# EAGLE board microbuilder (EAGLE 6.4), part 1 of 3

Size 273.6 x 738.6 mm. Coordinates in mm from the lower left corner, seen from the top.
Copper layers (1*16): Top 0.035mm / dielectric 1.5mm / Bottom 0.035mm
Design rules "default": minimum track width 10mil, minimum drill 24mil, track to track 8mil, track to pad 8mil, pad to pad 8mil, via to via 8mil, smd to smd 8mil, copper to edge 40mil, drill to drill 8mil, minimum pad ring 10mil, minimum via ring 8mil, stop-mask expansion 4mil, vias tented up to drill 0mil, thermal gap 10mil

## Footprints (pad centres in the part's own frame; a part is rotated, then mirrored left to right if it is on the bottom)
1X01_2MM = drill 0.8 pad 1.27: 1 0,0
1X01_2MM_OVAL = drill 0.8 pad 1.27 long: 1 0,0
1X01_OVAL = drill 1 pad 1.676 long: 1 0,0
1X01_ROUND = drill 1 pad 1.676: 1 0,0
1X02_OVAL = drill 1 long: 1 -1.27,0; 2 1.27,0
1X02_ROUND = drill 1 pad 1.676: 1 -1.27,0; 2 1.27,0
1X02_SMT = smd 1 x 3.5: 1 -1.27,1.27; 2 1.27,-1.27
1X03_1.0MM = smd 0.5 x 2.5: 1 -1,0; 2 0,0; 3 1,0
1X03_OVAL = drill 1 long: 1 -2.54,0; 2 0,0; 3 2.54,0
1X03_ROUND = drill 1 pad 1.676: 1 -2.54,0; 2 0,0; 3 2.54,0
1X03_ROUND_76 = drill 1 pad 1.93: 1 -2.54,0; 2 0,0; 3 2.54,0
1X03_SMT = smd 1 x 3.5: 1 -2.54,1.27; 2 0,-1.27; 3 2.54,1.27
1X04_1.0MM = smd 0.5 x 2.5: 1 -2,0; 2 -1,0; 3 0,0; 4 1,0
1X04_OVAL = drill 1 long: 1 -3.81,0; 2 -1.27,0; 3 1.27,0; 4 3.81,0
1X04_ROUND = drill 1 pad 1.676: 1 -3.81,0; 2 -1.27,0; 3 1.27,0; 4 3.81,0
1X04_ROUND_76 = drill 1 pad 1.93: 1 -3.81,0; 2 -1.27,0; 3 1.27,0; 4 3.81,0
1X04_SMT = smd 1 x 3: 1 -3.81,1.27; 2 -1.27,-1.27; 3 1.27,1.27; 4 3.81,-1.27
1X05_1.27MM = smd 0.5 x 2.5: 1 -2.54,0; 2 -1.27,0; 3 0,0; 4 1.27,0; 5 2.54,0
1X05_OVAL = drill 1 long: 1 -5.08,0; 2 -2.54,0; 3 0,0; 4 2.54,0; 5 5.08,0
1X05_ROUND = drill 1 pad 1.676: 1 -5.08,0; 2 -2.54,0; 3 0,0; 4 2.54,0; 5 5.08,0
1X05_ROUND_70 = drill 1 pad 1.778: 1 -5.08,0; 2 -2.54,0; 3 0,0; 4 2.54,0; 5 5.08,0
1X05_ROUND_76 = drill 1 pad 1.93: 1 -5.08,0; 2 -2.54,0; 3 0,0; 4 2.54,0; 5 5.08,0
1X05_SMT = smd 1 x 3.5: 1 -5.08,1.27; 2 -2.54,-1.27; 3 0,1.27; 4 2.54,-1.27; 5 5.08,1.27
1X06_OVAL = drill 1 long: 1 -6.35,0; 2 -3.81,0; 3 -1.27,0; 4 1.27,0; 5 3.81,0; 6 6.35,0
1X06_ROUND = drill 1 pad 1.676: 1 -6.35,0; 2 -3.81,0; 3 -1.27,0; 4 1.27,0; 5 3.81,0; 6 6.35,0
1X06_ROUND_70 = drill 1 pad 1.778: 1 -6.35,0; 2 -3.81,0; 3 -1.27,0; 4 1.27,0; 5 3.81,0; 6 6.35,0
1X06_ROUND_76 = drill 1 pad 1.93: 1 -6.35,0; 2 -3.81,0; 3 -1.27,0; 4 1.27,0; 5 3.81,0; 6 6.35,0
1X06_SMT = smd 1 x 3.5: 1 -6.35,1.27; 2 -3.81,-1.27; 3 -1.27,1.27; 4 1.27,-1.27; 5 3.81,1.27; 6 6.35,-1.27
1X07_OVAL = drill 1 long: 1 -7.62,0; 2 -5.08,0; 3 -2.54,0; 4 0,0; 5 2.54,0; 6 5.08,0; 7 7.62,0
1X07_ROUND = drill 1 pad 1.676: 1 -7.62,0; 2 -5.08,0; 3 -2.54,0; 4 0,0; 5 2.54,0; 6 5.08,0; 7 7.62,0
1X07_ROUND_70 = drill 1 pad 1.778: 1 -7.62,0; 2 -5.08,0; 3 -2.54,0; 4 0,0; 5 2.54,0; 6 5.08,0; 7 7.62,0
1X07_ROUND_76 = drill 1 pad 1.93: 1 -7.62,0; 2 -5.08,0; 3 -2.54,0; 4 0,0; 5 2.54,0; 6 5.08,0; 7 7.62,0
1X08_OVAL = drill 1 long: 1 -8.89,0; 2 -6.35,0; 3 -3.81,0; 4 -1.27,0; 5 1.27,0; 6 3.81,0; 7 6.35,0; 8 8.89,0
1X08_ROUND = drill 1 pad 1.676: 1 -8.89,0; 2 -6.35,0; 3 -3.81,0; 4 -1.27,0; 5 1.27,0; 6 3.81,0; 7 6.35,0; 8 8.89,0
1X08_ROUND_70 = drill 1 pad 1.778: 1 -8.89,0; 2 -6.35,0; 3 -3.81,0; 4 -1.27,0; 5 1.27,0; 6 3.81,0; 7 6.35,0; 8 8.89,0
1X08_ROUND_76 = drill 1 pad 1.93: 1 -8.89,0; 2 -6.35,0; 3 -3.81,0; 4 -1.27,0; 5 1.27,0; 6 3.81,0; 7 6.35,0; 8 8.89,0
1X09_OVAL = drill 1 long: 1 -10.16,0; 2 -7.62,0; 3 -5.08,0; 4 -2.54,0; 5 0,0; 6 2.54,0; 7 5.08,0; 8 7.62,0; 9 10.16,0
1X09_ROUND_70 = drill 1 pad 1.778: 1 -10.16,0; 2 -7.62,0; 3 -5.08,0; 4 -2.54,0; 5 0,0; 6 2.54,0; 7 5.08,0; 8 7.62,0; 9 10.16,0
1X09_ROUND_76 = drill 1 pad 1.93: 1 -10.16,0; 2 -7.62,0; 3 -5.08,0; 4 -2.54,0; 5 0,0; 6 2.54,0; 7 5.08,0; 8 7.62,0; 9 10.16,0
1X10_OVAL = drill 1 long: 1 -11.43,0; 2 -8.89,0; 3 -6.35,0; 4 -3.81,0; 5 -1.27,0; 6 1.27,0; 7 3.81,0; 8 6.35,0; 9 8.89,0; 10 11.43,0
1X10_ROUND = drill 1 pad 1.676: 1 -11.43,0; 2 -8.89,0; 3 -6.35,0; 4 -3.81,0; 5 -1.27,0; 6 1.27,0; 7 3.81,0; 8 6.35,0; 9 8.89,0; 10 11.43,0
1X10_ROUND70 = drill 1 pad 1.778: 1 -11.43,0; 2 -8.89,0; 3 -6.35,0; 4 -3.81,0; 5 -1.27,0; 6 1.27,0; 7 3.81,0; 8 6.35,0; 9 8.89,0; 10 11.43,0
1X10_ROUND_2MM = drill 1 pad 1.5: 1 -10,0; 2 -8,0; 3 -6,0; 4 -4,0; 5 -2,0; 6 0,0; 7 2,0; 8 4,0; 9 6,0; 10 8,0
1X10_ROUND_76 = drill 1 pad 1.93: 1 -11.43,0; 2 -8.89,0; 3 -6.35,0; 4 -3.81,0; 5 -1.27,0; 6 1.27,0; 7 3.81,0; 8 6.35,0; 9 8.89,0; 10 11.43,0
1X10_SMT = smd 1 x 3.5: 1 -11.43,1.27; 2 -8.89,-1.27; 3 -6.35,1.27; 4 -3.81,-1.27; 5 -1.27,1.27; 6 1.27,-1.27; 7 3.81,1.27; 8 6.35,-1.27; 9 8.89,1.27; 10 11.43,-1.27
1X11_ROUND = drill 1 pad 1.676: 1 -12.7,0; 2 -10.16,0; 3 -7.62,0; 4 -5.08,0; 5 -2.54,0; 6 0,0; 7 2.54,0; 8 5.08,0; 9 7.62,0; 10 10.16,0; 11 12.7,0
1X11_ROUND_76 = drill 1 pad 1.93: 1 -12.7,0; 2 -10.16,0; 3 -7.62,0; 4 -5.08,0; 5 -2.54,0; 6 0,0; 7 2.54,0; 8 5.08,0; 9 7.62,0; 10 10.16,0; 11 12.7,0
1X12_OVAL = drill 1 pad 1.676 long: 1 -13.97,0; 2 -11.43,0; 3 -8.89,0; 4 -6.35,0; 5 -3.81,0; 6 -1.27,0; 7 1.27,0; 8 3.81,0; 9 6.35,0; 10 8.89,0; 11 11.43,0; 12 13.97,0
1X12_ROUND = drill 1 pad 1.676: 1 -13.97,0; 2 -11.43,0; 3 -8.89,0; 4 -6.35,0; 5 -3.81,0; 6 -1.27,0; 7 1.27,0; 8 3.81,0; 9 6.35,0; 10 8.89,0; 11 11.43,0; 12 13.97,0
1X12_ROUND_76MIL = drill 1 pad 1.93: 1 -13.97,0; 2 -11.43,0; 3 -8.89,0; 4 -6.35,0; 5 -3.81,0; 6 -1.27,0; 7 1.27,0; 8 3.81,0; 9 6.35,0; 10 8.89,0; 11 11.43,0; 12 13.97,0
1X12_ROUND_80MIL = drill 1 pad 2.032: 1 -13.97,0; 2 -11.43,0; 3 -8.89,0; 4 -6.35,0; 5 -3.81,0; 6 -1.27,0; 7 1.27,0; 8 3.81,0; 9 6.35,0; 10 8.89,0; 11 11.43,0; 12 13.97,0
1X13_ROUND_70 = drill 1 pad 1.676: 1 -15.24,0; 2 -12.7,0; 3 -10.16,0; 4 -7.62,0; 5 -5.08,0; 6 -2.54,0; 7 0,0; 8 2.54,0; 9 5.08,0; 10 7.62,0; 11 10.16,0; 12 12.7,0; 13 15.24,0
1X15_ROUND_70 = drill 1 pad 1.676: 1 -17.78,0; 2 -15.24,0; 3 -12.7,0; 4 -10.16,0; 5 -7.62,0; 6 -5.08,0; 7 -2.54,0; 8 0,0; 9 2.54,0; 10 5.08,0; 11 7.62,0; 12 10.16,0; 13 12.7,0; 14 15.24,0; 15 17.78,0
1X16_2MM = drill 0.8 pad 1.27: P$1 -15,0; P$2 -13,0; P$3 -11,0; P$4 -9,0; P$5 -7,0; P$6 -5,0; P$7 -3,0; P$8 -1,0; P$9 1,0; P$10 3,0; P$11 5,0; P$12 7,0; P$13 9,0; P$14 11,0; P$15 13,0; P$16 15,0
1X16_2MM_OVAL = drill 0.8 pad 1.27 long: P$1 -15,0; P$2 -13,0; P$3 -11,0; P$4 -9,0; P$5 -7,0; P$6 -5,0; P$7 -3,0; P$8 -1,0; P$9 1,0; P$10 3,0; P$11 5,0; P$12 7,0; P$13 9,0; P$14 11,0; P$15 13,0; P$16 15,0
1X16_OVAL = drill 1 long: 1 -19.05,0; 2 -16.51,0; 3 -13.97,0; 4 -11.43,0; 5 -8.89,0; 6 -6.35,0; 7 -3.81,0; 8 -1.27,0; 9 1.27,0; 10 3.81,0; 11 6.35,0; 12 8.89,0; 13 11.43,0; 14 13.97,0; 15 16.51,0; 16 19.05,0
1X16_ROUND = drill 1 pad 1.676: 1 -19.05,0; 2 -16.51,0; 3 -13.97,0; 4 -11.43,0; 5 -8.89,0; 6 -6.35,0; 7 -3.81,0; 8 -1.27,0; 9 1.27,0; 10 3.81,0; 11 6.35,0; 12 8.89,0; 13 11.43,0; 14 13.97,0; 15 16.51,0; 16 19.05,0
1X17_ROUND70 = drill 1 pad 1.778: 1 -20.32,0; 2 -17.78,0; 3 -15.24,0; 4 -12.7,0; 5 -10.16,0; 6 -7.62,0; 7 -5.08,0; 8 -2.54,0; 9 0,0; 10 2.54,0; 11 5.08,0; 12 7.62,0; 13 10.16,0; 14 12.7,0; 15 15.24,0; 16 17.78,0; 17 20.32,0
1X20_ROUND = drill 1 pad 1.676: 1 -24.13,0; 2 -21.59,0; 3 -19.05,0; 4 -16.51,0; 5 -13.97,0; 6 -11.43,0; 7 -8.89,0; 8 -6.35,0; 9 -3.81,0; 10 -1.27,0; 11 1.27,0; 12 3.81,0; 13 6.35,0; 14 8.89,0; 15 11.43,0; 16 13.97,0; 17 16.51,0; 18 19.05,0; 19 21.59,0; 20 24.13,0
1X23_ROUND_70MIL = drill 1 pad 1.676: 1 -27.94,0; 2 -25.4,0; 3 -22.86,0; 4 -20.32,0; 5 -17.78,0; 6 -15.24,0; 7 -12.7,0; 8 -10.16,0; 9 -7.62,0; 10 -5.08,0; 11 -2.54,0; 12 0,0; 13 2.54,0; 14 5.08,0; 15 7.62,0; 16 10.16,0; 17 12.7,0; 18 15.24,0; 19 17.78,0; 20 20.32,0; 21 22.86,0; 22 25.4,0; 23 27.94,0
1X27_OVAL = drill 1 pad 1.676 long: 1 -34.29,0; 2 -31.75,0; 3 -29.21,0; 4 -26.67,0; 5 -24.13,0; 6 -21.59,0; 7 -19.05,0; 8 -16.51,0; 9 -13.97,0; 10 -11.43,0; 11 -8.89,0; 12 -6.35,0; 13 -3.81,0; 14 -1.27,0; 15 1.27,0; 16 3.81,0; 17 6.35,0; 18 8.89,0; 19 11.43,0; 20 13.97,0; 21 16.51,0; 22 19.05,0; 23 21.59,0; 24 24.13,0; 25 26.67,0; 26 29.21,0; 27 31.75,0
1X27_ROUND = drill 1 pad 1.676: 1 -33.02,0; 2 -30.48,0; 3 -27.94,0; 4 -25.4,0; 5 -22.86,0; 6 -20.32,0; 7 -17.78,0; 8 -15.24,0; 9 -12.7,0; 10 -10.16,0; 11 -7.62,0; 12 -5.08,0; 13 -2.54,0; 14 0,0; 15 2.54,0; 16 5.08,0; 17 7.62,0; 18 10.16,0; 19 12.7,0; 20 15.24,0; 21 17.78,0; 22 20.32,0; 23 22.86,0; 24 25.4,0; 25 27.94,0; 26 30.48,0; 27 33.02,0
1X28_OVAL = drill 1 pad 1.676 long: 1 -34.29,0; 2 -31.75,0; 3 -29.21,0; 4 -26.67,0; 5 -24.13,0; 6 -21.59,0; 7 -19.05,0; 8 -16.51,0; 9 -13.97,0; 10 -11.43,0; 11 -8.89,0; 12 -6.35,0; 13 -3.81,0; 14 -1.27,0; 15 1.27,0; 16 3.81,0; 17 6.35,0; 18 8.89,0; 19 11.43,0; 20 13.97,0; 21 16.51,0; 22 19.05,0; 23 21.59,0; 24 24.13,0; 25 26.67,0; 26 29.21,0; 27 31.75,0; 28 34.29,0
2X03_ROUND_70MIL = drill 1 pad 1.778: 1 -2.54,1.27; 2 -2.54,-1.27; 3 0,1.27; 4 0,-1.27; 5 2.54,1.27; 6 2.54,-1.27
2X05 = drill 1 square: 1 -5.08,-1.27 | drill 1: 2 -5.08,1.27; 3 -2.54,-1.27; 4 -2.54,1.27; 5 0,-1.27; 6 0,1.27; 7 2.54,-1.27; 8 2.54,1.27; 9 5.08,-1.27; 10 5.08,1.27
2X05_1.27MM_SMT = smd 0.65 x 2.6: 1 -2.54,-1.85; 2 -2.54,1.85; 3 -1.27,-1.85; 4 -1.27,1.85; 5 0,-1.85; 6 0,1.85; 7 1.27,-1.85; 8 1.27,1.85; 9 2.54,-1.85; 10 2.54,1.85
2X07 = drill 1 square: 1 -7.62,-1.27 | drill 1: 2 -7.62,1.27; 3 -5.08,-1.27; 4 -5.08,1.27; 5 -2.54,-1.27; 6 -2.54,1.27; 7 0,-1.27; 8 0,1.27; 9 2.54,-1.27; 10 2.54,1.27; 11 5.08,-1.27; 12 5.08,1.27; 13 7.62,-1.27; 14 7.62,1.27
2X08 = drill 1 square: 1 -8.89,-1.27 | drill 1 pad 1.676: 2 -8.89,1.27; 3 -6.35,-1.27; 4 -6.35,1.27; 5 -3.81,-1.27; 6 -3.81,1.27; 7 -1.27,-1.27; 8 -1.27,1.27; 9 1.27,-1.27; 10 1.27,1.27; 11 3.81,-1.27; 12 3.81,1.27; 13 6.35,-1.27; 14 6.35,1.27; 15 8.89,-1.27; 16 8.89,1.27
2X10 = drill 1 square: 1 -11.43,-1.27 | drill 1: 2 -11.43,1.27; 3 -8.89,-1.27; 4 -8.89,1.27; 5 -6.35,-1.27; 6 -6.35,1.27; 7 -3.81,-1.27; 8 -3.81,1.27; 9 -1.27,-1.27; 10 -1.27,1.27; 11 1.27,-1.27; 12 1.27,1.27; 13 3.81,-1.27; 14 3.81,1.27; 15 6.35,-1.27; 16 6.35,1.27; 17 8.89,-1.27; 18 8.89,1.27; 19 11.43,-1.27; 20 11.43,1.27
2X13 = drill 1 pad 1.676 square: 1 -15.24,-1.27 | drill 1 pad 1.676: 2 -15.24,1.27; 3 -12.7,-1.27; 4 -12.7,1.27; 5 -10.16,-1.27; 6 -10.16,1.27; 7 -7.62,-1.27; 8 -7.62,1.27; 9 -5.08,-1.27; 10 -5.08,1.27; 11 -2.54,-1.27; 12 -2.54,1.27; 13 0,-1.27; 14 0,1.27; 15 2.54,-1.27; 16 2.54,1.27; 17 5.08,-1.27; 18 5.08,1.27; 19 7.62,-1.27; 20 7.62,1.27; 21 10.16,-1.27; 22 10.16,1.27; 23 12.7,-1.27; 24 12.7,1.27; 25 15.24,-1.27; 26 15.24,1.27
2X15 = drill 1 pad 1.676 square: 1 -17.78,-1.27 | drill 1 pad 1.676: 2 -17.78,1.27; 3 -15.24,-1.27; 4 -15.24,1.27; 5 -12.7,-1.27; 6 -12.7,1.27; 7 -10.16,-1.27; 8 -10.16,1.27; 9 -7.62,-1.27; 10 -7.62,1.27; 11 -5.08,-1.27; 12 -5.08,1.27; 13 -2.54,-1.27; 14 -2.54,1.27; 15 0,-1.27; 16 0,1.27; 17 2.54,-1.27; 18 2.54,1.27; 19 5.08,-1.27; 20 5.08,1.27; 21 7.62,-1.27; 22 7.62,1.27; 23 10.16,-1.27; 24 10.16,1.27; 25 12.7,-1.27; 26 12.7,1.27; 27 15.24,-1.27; 28 15.24,1.27; 29 17.78,-1.27; 30 17.78,1.27
2X16 = drill 1 square: 1 -19.05,-1.27 | drill 1: 2 -19.05,1.27; 3 -16.51,-1.27; 4 -16.51,1.27; 5 -13.97,-1.27; 6 -13.97,1.27; 7 -11.43,-1.27; 8 -11.43,1.27; 9 -8.89,-1.27; 10 -8.89,1.27; 11 -6.35,-1.27; 12 -6.35,1.27; 13 -3.81,-1.27; 14 -3.81,1.27; 15 -1.27,-1.27; 16 -1.27,1.27; 17 1.27,-1.27; 18 1.27,1.27; 19 3.81,-1.27; 20 3.81,1.27; 21 6.35,-1.27; 22 6.35,1.27; 23 8.89,-1.27; 24 8.89,1.27; 25 11.43,-1.27; 26 11.43,1.27; 27 13.97,-1.27; 28 13.97,1.27; 29 16.51,-1.27; 30 16.51,1.27; 31 19.05,-1.27; 32 19.05,1.27
2X23 = drill 1 square: 1 -27.94,-1.27 | drill 1: 2 -27.94,1.27; 3 -25.4,-1.27; 4 -25.4,1.27; 5 -22.86,-1.27; 6 -22.86,1.27; 7 -20.32,-1.27; 8 -20.32,1.27; 9 -17.78,-1.27; 10 -17.78,1.27; 11 -15.24,-1.27; 12 -15.24,1.27; 13 -12.7,-1.27; 14 -12.7,1.27; 15 -10.16,-1.27; 16 -10.16,1.27; 17 -7.62,-1.27; 18 -7.62,1.27; 19 -5.08,-1.27; 20 -5.08,1.27; 21 -2.54,-1.27; 22 -2.54,1.27; 23 0,-1.27; 24 0,1.27; 25 2.54,-1.27; 26 2.54,1.27; 27 5.08,-1.27; 28 5.08,1.27; 29 7.62,-1.27; 30 7.62,1.27; 31 10.16,-1.27; 32 10.16,1.27; 33 12.7,-1.27; 34 12.7,1.27; 35 15.24,-1.27; 36 15.24,1.27; 37 17.78,-1.27; 38 17.78,1.27; 39 20.32,-1.27; 40 20.32,1.27; 41 22.86,-1.27; 42 22.86,1.27; 43 25.4,-1.27; 44 25.4,1.27; 45 27.94,-1.27; 46 27.94,1.27
3X04 = drill 1 pad 1.778 square: 1 -3.81,-2.54 | drill 1 pad 1.778: 2 -3.81,0; 3 -3.81,2.54; 4 -1.27,-2.54; 5 -1.27,0; 6 -1.27,2.54; 7 1.27,-2.54; 8 1.27,0; 9 1.27,2.54; 10 3.81,-2.54; 11 3.81,0; 12 3.81,2.54
3X08 = drill 1 pad 1.778 square: 1 -8.89,-2.54 | drill 1 pad 1.778: 2 -8.89,0; 3 -8.89,2.54; 4 -6.35,-2.54; 5 -6.35,0; 6 -6.35,2.54; 7 -3.81,-2.54; 8 -3.81,0; 9 -3.81,2.54; 10 -1.27,-2.54; 11 -1.27,0; 12 -1.27,2.54; 13 1.27,-2.54; 14 1.27,0; 15 1.27,2.54; 16 3.81,-2.54; 17 3.81,0; 18 3.81,2.54; 19 6.35,-2.54; 20 6.35,0; 21 6.35,2.54; 22 8.89,-2.54; 23 8.89,0; 24 8.89,2.54
4UCONN_05550 = drill 1.8 pad 2.54: 1 1.2,-0.9; 4 13,-0.9; 5 3.6,1.1 | drill 1.8 pad 2.4: 2 7.3,-0.9 | drill 1.7 pad 2.184: 3 9.3,1.1
4UCONN_19269 = smd 2 x 2.5: 1 2.5,-3.5; 2 11.7,-3.5; 3 4.3,3.5 | smd 2.5 x 2: 4 15.8,0.75 | smd 1.2 x 2.5: 5 1.5,3.5 | hole 2: 3.5,0; 10.5,0
4UCONN_19621 = smd 1.5 x 2.5: 1-GND 2.8,-3.3; 2-TIP 9.3,3.4; 3-OUTER_SLEEVE 5.5,-3.3; 6-OUTER_SLEEVE_BREAK 10.6,-3.3 | smd 1.5 x 3.4: 4-INNER_SLEEVE 2.8,2.9; 5-TIP_BREAK 11.5,2.9 | hole 1.3: 10.5,0
4UCONN_19621_SPARK = smd 1.5 x 2.5: 1-GND 2.8,-3.6; 2-TIP 9.3,3.6; 3-OUTER_SLEEVE 5.5,-3.6; 6-OUTER_SLEEVE_BREAK 10.6,-3.6 | smd 1.5 x 3.4: 4-INNER_SLEEVE 2.8,3.2; 5-TIP_BREAK 11.5,3.2 | hole 1.3: 10.5,0
32QN2 = smd 0.7 x 0.25: 1 -2.45,1.75; 2 -2.45,1.25; 3 -2.45,0.75; 4 -2.45,0.25; 5 -2.45,-0.25; 6 -2.45,-0.75; 7 -2.45,-1.25; 8 -2.45,-1.75; 17 2.45,-1.75; 18 2.45,-1.25; 19 2.45,-0.75; 20 2.45,-0.25; 21 2.45,0.25; 22 2.45,0.75; 23 2.45,1.25; 24 2.45,1.75 | smd 0.25 x 0.7: 9 -1.75,-2.45; 10 -1.25,-2.45; 11 -0.75,-2.45; 12 -0.25,-2.45; 13 0.25,-2.45; 14 0.75,-2.45; 15 1.25,-2.45; 16 1.75,-2.45; 25 1.75,2.45; 26 1.25,2.45; 27 0.75,2.45; 28 0.25,2.45; 29 -0.25,2.45; 30 -0.75,2.45; 31 -1.25,2.45; 32 -1.75,2.45 | smd 3.3 x 3.3: 33 0,0
869MHZANTENNA = smd 2 x 2.5: P$1 -12.7,-6.858; P$2 -7.62,-6.858; P$3 -2.54,-6.858; P$4 2.54,-6.858; P$5 7.62,-6.858; P$6 12.7,-6.858
0402 = smd 0.7 x 0.9: 1 -0.65,0; 2 0.65,0
0603 = smd 1.1 x 1: 1 -0.85,0; 2 0.85,0
0603-MINI = smd 0.9 x 0.9: 1 -0.75,0; 2 0.75,0
0805 = smd 1.3 x 1.5: 1 -0.95,0; 2 0.95,0
0805-THM = drill 0.813 pad 1.676 octagon: 1 -5.08,0; 2 5.08,0
0805_NOTHERMALS = smd 1.3 x 1.5: 1 -0.95,0; 2 0.95,0
1206 = smd 1.6 x 1.8: 1 -1.4,0; 2 1.4,0
2012 = smd 1.8 x 2.7: 1 -2.2,0; 2 2.2,0
2512 = smd 1.8 x 3.2: 1 -2.8,0; 2 2.8,0
ADBM-A350 = smd 0.3 x 0.8: 1 -2.4,16.38; 2 -2.1,19.18; 3 -1.8,16.38; 4 -1.5,19.18; 5 -1.2,16.38; 6 -0.9,19.18; 7 -0.6,16.38; 8 -0.3,19.18; 9 0,16.38; 10 0.3,19.18; 11 0.6,16.38; 12 0.9,19.18; 13 1.2,16.38; 14 1.5,19.18; 15 1.8,16.38; 16 2.1,19.18; 17 2.4,16.38
ANT_868MHZ_SPLATCH = smd 2 x 2.5: GND1 -7.62,0; GND2 -2.54,0; GND3 2.54,0; GND4 7.62,0; GND5 12.7,0; MICROSTRIP -12.7,0
ARDUINO = drill 1 pad 1.676 octagon: 3V 36.068,2.54; 5V 38.608,2.54; A0 51.308,2.54; A1 53.848,2.54; A2 56.388,2.54; A3 58.928,2.54; A4 61.468,2.54; A5 64.008,2.54; AREF 24.384,50.8; D0 63.881,50.8; D1 61.341,50.8; D2 58.801,50.8; D3 56.261,50.8; D4 53.721,50.8; D5 51.181,50.8; D6 48.641,50.8; D7 46.101,50.8; D8 42.164,50.8; D9 39.624,50.8; D10 37.084,50.8; D11 34.544,50.8; D12 32.004,50.8; D13 29.464,50.8; GND 26.924,50.8; GND1 43.688,2.54; GND2 41.148,2.54; RESET 33.528,2.54; VIN 46.228,2.54 | hole 3.2: 15.758,50.754 | hole 2.2: 66.558,35.514
ARDUINO-NODIM = drill 1 pad 1.676 octagon: 3V 36.068,2.54; 5V 38.608,2.54; A0 51.308,2.54; A1 53.848,2.54; A2 56.388,2.54; A3 58.928,2.54; A4 61.468,2.54; A5 64.008,2.54; AREF 24.384,50.8; D0 63.881,50.8; D1 61.341,50.8; D2 58.801,50.8; D3 56.261,50.8; D4 53.721,50.8; D5 51.181,50.8; D6 48.641,50.8; D7 46.101,50.8; D8 42.164,50.8; D9 39.624,50.8; D10 37.084,50.8; D11 34.544,50.8; D12 32.004,50.8; D13 29.464,50.8; GND 26.924,50.8; GND1 43.688,2.54; GND2 41.148,2.54; RESET 33.528,2.54; VIN 46.228,2.54
ARDUINO-NOHOLE = drill 1 pad 1.676 octagon: 3V 36.068,2.54; 5V 38.608,2.54; A0 51.308,2.54; A1 53.848,2.54; A2 56.388,2.54; A3 58.928,2.54; A4 61.468,2.54; A5 64.008,2.54; AREF 24.384,50.8; D0 63.881,50.8; D1 61.341,50.8; D2 58.801,50.8; D3 56.261,50.8; D4 53.721,50.8; D5 51.181,50.8; D6 48.641,50.8; D7 46.101,50.8; D8 42.164,50.8; D9 39.624,50.8; D10 37.084,50.8; D11 34.544,50.8; D12 32.004,50.8; D13 29.464,50.8; GND 26.924,50.8; GND1 43.688,2.54; GND2 41.148,2.54; RESET 33.528,2.54; VIN 46.228,2.54
ARDUINOR3 = drill 1 pad 1.676 octagon: 3V 35.56,2.54; 5V 38.1,2.54; A0 50.8,2.54; A1 53.34,2.54; A2 55.88,2.54; A3 58.42,2.54; A4 60.96,2.54; A5 63.5,2.54; AREF 23.876,50.8; D0 63.5,50.8; D1 60.96,50.8; D2 58.42,50.8; D3 55.88,50.8; D4 53.34,50.8; D5 50.8,50.8; D6 48.26,50.8; D7 45.72,50.8; D8 41.656,50.8; D9 39.116,50.8; D10 36.576,50.8; D11 34.036,50.8; D12 31.496,50.8; D13 28.956,50.8; GND 26.416,50.8; GND1 43.18,2.54; GND2 40.64,2.54; IOREF 30.48,2.54; RESERVED 27.94,2.54; RESET 33.02,2.54; SCL 18.796,50.8; SDA 21.336,50.8; VIN 45.72,2.54
ARDUINOR3-BPLACE = drill 1 pad 1.676 octagon: 3V 35.56,2.54; 5V 38.1,2.54; A0 50.8,2.54; A1 53.34,2.54; A2 55.88,2.54; A3 58.42,2.54; A4 60.96,2.54; A5 63.5,2.54; AREF 23.876,50.8; D0 63.5,50.8; D1 60.96,50.8; D2 58.42,50.8; D3 55.88,50.8; D4 53.34,50.8; D5 50.8,50.8; D6 48.26,50.8; D7 45.72,50.8; D8 41.656,50.8; D9 39.116,50.8; D10 36.576,50.8; D11 34.036,50.8; D12 31.496,50.8; D13 28.956,50.8; GND 26.416,50.8; GND1 43.18,2.54; GND2 40.64,2.54; IOREF 30.48,2.54; RESERVED 27.94,2.54; RESET 33.02,2.54; SCL 18.796,50.8; SDA 21.336,50.8; VIN 45.72,2.54
ARDUINOR3-NODIM = drill 1 pad 1.676 octagon: 3V 35.56,2.54; 5V 38.1,2.54; A0 50.8,2.54; A1 53.34,2.54; A2 55.88,2.54; A3 58.42,2.54; A4 60.96,2.54; A5 63.5,2.54; AREF 23.876,50.8; D0 63.5,50.8; D1 60.96,50.8; D2 58.42,50.8; D3 55.88,50.8; D4 53.34,50.8; D5 50.8,50.8; D6 48.26,50.8; D7 45.72,50.8; D8 41.656,50.8; D9 39.116,50.8; D10 36.576,50.8; D11 34.036,50.8; D12 31.496,50.8; D13 28.956,50.8; GND 26.416,50.8; GND1 43.18,2.54; GND2 40.64,2.54; IOREF 30.48,2.54; RESERVED 27.94,2.54; RESET 33.02,2.54; SCL 18.796,50.8; SDA 21.336,50.8; VIN 45.72,2.54
BALUN0603 = smd 0.2 x 0.5: 1 0.5,0.5; 2 0,0.5; 3 -0.5,0.5; 4 -0.5,-0.5; 5 0,-0.5; 6 0.5,-0.5
BALUN0805 = smd 0.3 x 0.7: 1 0.65,0.65; 2 0,0.65; 3 -0.65,0.65; 4 -0.65,-0.65; 5 0,-0.65; 6 0.65,-0.65
BALUN1206 = smd 0.55 x 0.85: P$1 1,0.9; P$2 0,0.9; P$3 -1,0.9; P$4 -1,-0.9; P$5 0,-0.9; P$6 1,-0.9
BEAGLEBONE_SHIELD = drill 1 square: 1 4.445,19.05; 47 52.705,19.05 | drill 1: 2 1.905,19.05; 3 4.445,21.59; 4 1.905,21.59; 5 4.445,24.13; 6 1.905,24.13; 7 4.445,26.67; 8 1.905,26.67; 9 4.445,29.21; 10 1.905,29.21; 11 4.445,31.75; 12 1.905,31.75; 13 4.445,34.29; 14 1.905,34.29; 15 4.445,36.83; 16 1.905,36.83; 17 4.445,39.37; 18 1.905,39.37; 19 4.445,41.91; 20 1.905,41.91; 21 4.445,44.45; 22 1.905,44.45; 23 4.445,46.99; 24 1.905,46.99; 25 4.445,49.53; 26 1.905,49.53; 27 4.445,52.07; 28 1.905,52.07; 29 4.445,54.61; 30 1.905,54.61; 31 4.445,57.15; 32 1.905,57.15; 33 4.445,59.69; 34 1.905,59.69; 35 4.445,62.23; 36 1.905,62.23; 37 4.445,64.77; 38 1.905,64.77; 39 4.445,67.31; 40 1.905,67.31; 41 4.445,69.85; 42 1.905,69.85; 43 4.445,72.39; 44 1.905,72.39; 45 4.445,74.93; 46 1.905,74.93; 48 50.165,19.05; 49 52.705,21.59; 50 50.165,21.59; 51 52.705,24.13; 52 50.165,24.13; 53 52.705,26.67; 54 50.165,26.67; 55 52.705,29.21; 56 50.165,29.21; 57 52.705,31.75; 58 50.165,31.75; 59 52.705,34.29; 60 50.165,34.29; 61 52.705,36.83; 62 50.165,36.83; 63 52.705,39.37; 64 50.165,39.37; 65 52.705,41.91; 66 50.165,41.91; 67 52.705,44.45; 68 50.165,44.45; 69 52.705,46.99; 70 50.165,46.99; 71 52.705,49.53; 72 50.165,49.53; 73 52.705,52.07; 74 50.165,52.07; 75 52.705,54.61; 76 50.165,54.61; 77 52.705,57.15; 78 50.165,57.15; 79 52.705,59.69; 80 50.165,59.69; 81 52.705,62.23; 82 50.165,62.23; 83 52.705,64.77; 84 50.165,64.77; 85 52.705,67.31; 86 50.165,67.31; 87 52.705,69.85; 88 50.165,69.85; 89 52.705,72.39; 90 50.165,72.39; 91 52.705,74.93; 92 50.165,74.93
BLUETOOTH_MODULE = smd 2.5 x 0.9: 1 -6.9,6.35; 2 -6.9,4.85; 3 -6.9,3.35; 4 -6.9,1.85; 5 -6.9,0.35; 6 -6.9,-1.15; 7 -6.9,-2.65; 8 -6.9,-4.15; 9 -6.9,-5.65; 10 -6.9,-7.15; 11 -6.9,-8.65; 12 -6.9,-10.15; 13 -6.9,-11.65; 22 6.9,-11.65; 23 6.9,-10.15; 24 6.9,-8.65; 25 6.9,-7.15; 26 6.9,-5.65; 27 6.9,-4.15; 28 6.9,-2.65; 29 6.9,-1.15; 30 6.9,0.35; 31 6.9,1.85; 32 6.9,3.35; 33 6.9,4.85; 34 6.9,6.35 | smd 0.9 x 2.5: 14 -5.25,-13.83; 15 -3.75,-13.83; 16 -2.25,-13.83; 17 -0.75,-13.83; 18 0.75,-13.83; 19 2.25,-13.83; 20 3.75,-13.83; 21 5.25,-13.83
BMC050 = smd 0.6 x 0.25: 1 -1.2,0.5; 2 -1.2,0; 3 -1.2,-0.5; 9 1.2,-0.5; 10 1.2,0; 11 1.2,0.5 | smd 0.28 x 0.65: 4 -1,-1.2; 5 -0.5,-1.2; 6 0,-1.2; 7 0.5,-1.2; 8 1,-1.2; 12 1,1.2; 13 0.5,1.2; 14 0,1.2; 15 -0.5,1.2; 16 -1,1.2
BMC050_EXTENDED = smd 1.1 x 0.25: 1 -1.45,0.5; 2 -1.45,0; 3 -1.45,-0.5; 9 1.45,-0.5; 10 1.45,0; 11 1.45,0.5 | smd 0.28 x 1.15: 4 -1,-1.45; 5 -0.5,-1.45; 6 0,-1.45; 7 0.5,-1.45; 8 1,-1.45; 12 1,1.45; 13 0.5,1.45; 14 0,1.45; 15 -0.5,1.45; 16 -1,1.45
BMP085 = smd 1.67 x 0.8: P$1 -2.065,1.27; P$2 -2.065,0; P$3 -2.065,-1.27; P$5 2.065,-1.27; P$6 2.065,0; P$7 2.065,1.27 | smd 0.8 x 1.67: P$4 0,-2.065 | smd 0.8 x 2.5: P$8 0,1.65
BREAKOUT_SOIC8 = smd 0.66 x 3.81: 1 -1.905,-4.14; 2 -0.635,-4.14; 3 0.635,-4.14; 4 1.905,-4.14; 5 1.905,4.14; 6 0.635,4.14; 7 -0.635,4.14; 8 -1.905,4.14
BREAKOUT_SOIC24 = smd 0.66 x 3.81: 1 -6.985,-4.14; 2 -5.715,-4.14; 3 -4.445,-4.14; 4 -3.175,-4.14; 5 -1.905,-4.14; 6 -0.635,-4.14; 7 0.635,-4.14; 8 1.905,-4.14; 9 3.175,-4.14; 10 4.445,-4.14; 11 5.715,-4.14; 12 6.985,-4.14; 13 6.985,4.14; 14 5.715,4.14; 15 4.445,4.14; 16 3.175,4.14; 17 1.905,4.14; 18 0.635,4.14; 19 -0.635,4.14; 20 -1.905,4.14; 21 -3.175,4.14; 22 -4.445,4.14; 23 -5.715,4.14; 24 -6.985,4.14
BREAKOUT_SOT23-6 = smd 0.55 x 1.6: 1 -0.95,-1.5; 2 0,-1.5; 3 0.95,-1.5; 4 0.95,1.5; 5 0,1.5; 6 -0.95,1.5
BTL221722-276L = smd 0.5 x 3: 1 -5.2,-16.44; 2 -4.4,-16.44; 3 -3.6,-16.44; 4 -2.8,-16.44; 5 -2,-16.44; 6 -1.2,-16.44; 7 -0.4,-16.44; 8 0.4,-16.44; 9 1.2,-16.44; 10 2,-16.44; 11 2.8,-16.44; 12 3.6,-16.44; 13 4.4,-16.44; 14 5.2,-16.44 | hole 1: -15,-19.06; 15,-19.06 | hole 1.8: -19.75,-31.5; 19.75,-31.5; 19.75,23; -19.75,23
BTN_EVQPQ_4.5MM = smd 0.9 x 1: A -1.95,1.925; B 1.95,1.925; C -1.95,-1.925; D 1.95,-1.925
BTN_KMR2_4.6X2.8 = smd 0.9 x 1: A 2.05,0.8; A' -2.05,0.8; B 2.05,-0.8; B' -2.05,-0.8
C707_10M006_512_2 = smd 1.7 x 1.3: C1 -12.85,-3.915; C2 -12.85,-1.375; C3 -12.85,1.165; C5 12.85,-3.915; C6 12.85,-1.375; C7 12.85,1.165
CELEC_3.5MM_8MM = drill 0.813 pad 1.6: + -1.778,0 | drill 0.813 pad 1.6 octagon: - 1.778,0
CELEC_3.5MM_10MM = drill 0.813 pad 1.6: + -1.778,0 | drill 0.813 pad 1.6 octagon: - 1.778,0
CFAF240320K-T-TS = smd 0.4 x 2: P$1 0,0; P$2 0.8,0; P$3 1.6,0; P$4 2.4,0; P$5 3.2,0; P$6 4,0; P$7 4.8,0; P$8 5.6,0; P$9 6.4,0; P$10 7.2,0; P$11 8,0; P$12 8.8,0; P$13 9.6,0; P$14 10.4,0; P$15 11.2,0; P$16 12,0; P$17 12.8,0; P$18 13.6,0; P$19 14.4,0; P$20 15.2,0; P$21 16,0; P$22 16.8,0; P$23 17.6,0; P$24 18.4,0; P$25 19.2,0; P$26 20,0; P$27 20.8,0; P$28 21.6,0; P$29 22.4,0; P$30 23.2,0; P$31 24,0; P$32 24.8,0; P$33 25.6,0; P$34 26.4,0; P$35 27.2,0; P$36 28,0; P$37 28.8,0 | hole 1: -1.725,0; 30.53,0
CHIPLED_0603 = smd 0.8 x 0.8: A 0,-0.75; C 0,0.75
CHIPLED_0603_NOOUTLINE = smd 0.8 x 0.8: A 0,-0.75; C 0,0.75
CHIPLED_0805 = smd 1.2 x 1.2: A 0,-1.05; C 0,1.05
CHIPLED_0805_NOOUTLINE = smd 1.2 x 1.2: A 0,-1.05; C 0,1.05
CHIPLED_1206 = smd 1.5 x 1.5: A 0,-1.496; C 0,1.496
CORTEXM3_SWD10_MOLEX = drill 1: 1 -5.08,-1.27 | drill 1 octagon: 2 -5.08,1.27; 3 -2.54,-1.27; 4 -2.54,1.27; 5 0,-1.27; 6 0,1.27; 7 2.54,-1.27; 8 2.54,1.27; 9 5.08,-1.27; 10 5.08,1.27
CR1220 = smd 3.2 x 3.2: +$1 -8.225,0; +$2 8.225,0 | smd 6.35 x 6.35: - 0,0
CR2032 = drill 0.9: + 10,0; - -10,0
CRYSTAL_2.5X2 = smd 0.9 x 0.8: 1 -0.825,-0.625; 2 0.825,-0.625; 3 0.825,0.625; 4 -0.825,0.625
CRYSTAL_3.2X2.5 = smd 1.4 x 1.2: 1 -1.1,-0.8; 2 1.1,0.8; GND1 -1.1,0.8; GND2 1.1,-0.8
CRYSTAL_4.9X1.8 = smd 1.3 x 2.2: 1 -2.1,0; 2 2.1,0
CRYSTAL_8X3.8 = smd 1.3 x 1.9: P$1 -2.75,-1.6; P$2 2.75,-1.6; P$3 2.75,1.6; P$4 -2.75,1.6
CRYSTAL_CYL_2X6MM_SMT = smd 2.5 x 1: 1 2.125,1.27; 2 2.125,-1.27 | smd 6 x 2.5: CYLINDER -3.875,0
DCJACK_1.3MM_PTH = drill 1.3 long: GND 0,6; GNDBREAK 2.8,8.3; PWR 0,10.9
DCJACK_2MM_PTH = drill 2.8: GND 0,7.35; GNDBREAK 4.8,10.75 | drill 3.2: PWR 0,13.6
DCJACK_2MM_SMT = smd 2.4 x 2: GND 0,-5.5; GNDBREAK 6.2,-5.5; PWR 0,5.5; PWR2 6.2,5.5 | hole 1.6: 0,0 | hole 1.8: 4.5,0
DFN10_3X3MM = smd 0.25 x 0.8: 1 -1,-1.5; 2 -0.5,-1.5; 3 0,-1.5; 4 0.5,-1.5; 5 1,-1.5; 6 1,1.5; 7 0.5,1.5; 8 0,1.5; 9 -0.5,1.5; 10 -1,1.5 | smd 2.35 x 1.58: GND 0,0
DFN14_4X3MM = smd 0.25 x 0.8: 1 -1.5,-1.5; 2 -1,-1.5; 3 -0.5,-1.5; 4 0,-1.5; 5 0.5,-1.5; 6 1,-1.5; 7 1.5,-1.5; 8 1.5,1.5; 9 1,1.5; 10 0.5,1.5; 11 0,1.5; 12 -0.5,1.5; 13 -1,1.5; 14 -1.5,1.5 | smd 3.3 x 1.7: THERM 0,0
DIL08 = drill 0.813 long: 1 -3.81,-3.81; 2 -1.27,-3.81; 3 1.27,-3.81; 4 3.81,-3.81; 5 3.81,3.81; 6 1.27,3.81; 7 -1.27,3.81; 8 -3.81,3.81
DIL28_600MIL = drill 0.813 long: 1 -16.51,-7.75; 2 -13.97,-7.75; 3 -11.43,-7.75; 4 -8.89,-7.75; 5 -6.35,-7.75; 6 -3.81,-7.75; 7 -1.27,-7.75; 8 1.27,-7.75; 9 3.81,-7.75; 10 6.35,-7.75; 11 8.89,-7.75; 12 11.43,-7.75; 13 13.97,-7.75; 14 16.51,-7.75; 15 16.51,7.75; 16 13.97,7.75; 17 11.43,7.75; 18 8.89,7.75; 19 6.35,7.75; 20 3.81,7.75; 21 1.27,7.75; 22 -1.27,7.75; 23 -3.81,7.75; 24 -6.35,7.75; 25 -8.89,7.75; 26 -11.43,7.75; 27 -13.97,7.75; 28 -16.51,7.75
DIL40_0.9 = drill 1 pad 1.397 octagon: 1 -22.86,-11.43; 2 -20.32,-11.43; 3 -17.78,-11.43; 4 -15.24,-11.43; 5 -12.7,-11.43; 6 -10.16,-11.43; 7 -7.62,-11.43; 8 -5.08,-11.43; 9 -2.54,-11.43; 10 0,-11.43; 11 2.54,-11.43; 12 5.08,-11.43; 13 7.62,-11.43; 14 10.16,-11.43; 15 12.7,-11.43; 16 15.24,-11.43; 17 17.78,-11.43; 18 20.32,-11.43; 19 22.86,-11.43; 20 25.4,-11.43; 21 25.4,11.43; 22 22.86,11.43; 23 20.32,11.43; 24 17.78,11.43; 25 15.24,11.43; 26 12.7,11.43; 27 10.16,11.43; 28 7.62,11.43; 29 5.08,11.43; 30 2.54,11.43; 31 0,11.43; 32 -2.54,11.43; 33 -5.08,11.43; 34 -7.62,11.43; 35 -10.16,11.43; 36 -12.7,11.43; 37 -15.24,11.43; 38 -17.78,11.43; 39 -20.32,11.43; 40 -22.86,11.43
DIPSWITCH_2PIN = smd 1.1 x 2: 1A -1.27,-4.4; 1B -1.27,4.4; 2A 1.27,-4.4; 2B 1.27,4.4
DO-1N4148 = drill 0.9: A -3.81,0; C 3.81,0
DPDT_SMT_JS202011SCQN = smd 1.2 x 2.5: P$1 -2.5,-4; P$2 0,-4; P$3 2.5,-4; P$4 2.5,4; P$5 0,4; P$6 -2.5,4
EIA3216-18/A-R = smd 1.95 x 1.5: + 1.375,0; - -1.375,0
EIA3216-18/A-W = smd 2.15 x 1.8: + 1.475,0; - -1.475,0
EIA3528-21/B-R = smd 1.95 x 2.5: + 1.525,0; - -1.525,0
EIA3528-21/B-W = smd 2.15 x 1.8: + 1.625,0; - -1.625,0
EIA6032-28/C-R = smd 2.55 x 2.5: + 2.525,0; - -2.525,0
EIA6032-28/C-W = smd 2.75 x 1.8: + 2.625,0; - -2.625,0
EIA7343-31/D-R = smd 2.55 x 2.7: + 3.175,0; - -3.175,0
EIA7343-31/D-W = smd 2.95 x 2.7: + 3.375,0; - -3.375,0
EINK_10BAR = smd 2 x 0.25: P$1 0,1.4; P$2 0,1.9; P$3 0,2.4; P$4 0,2.9; P$5 0,3.4; P$6 0,3.9; P$7 0,4.4; P$8 0,4.9; P$9 0,5.4; P$10 0,5.9; P$11 0,6.4; P$12 0,6.9
ENCLOSURE_SS125 = hole 3.2: 4.5,93; 64.5,93; 4.5,8; 64.5,8; 64.5,50.5; 4.5,50.5
EVQ-Q2 = smd 3.2 x 1.2: A -3.4,-2; A' 3.4,-2; B -3.4,2; B' 3.4,2
FGPMMOPA6B = smd 3 x 1: P$1 -8.5,6.75; P$2 -8.5,5.25; P$3 -8.5,3.75; P$4 -8.5,2.25; P$5 -8.5,0.75; P$6 -8.5,-0.75; P$7 -8.5,-2.25; P$8 -8.5,-3.75; P$9 -8.5,-5.25; P$10 -8.5,-6.75; P$11 8.5,6.75; P$12 8.5,-6.75 | hole 3: 0.5,0.85
FGPMMOPA6C = smd 3 x 1: P$1 -8.5,6.75; P$2 -8.5,5.25; P$3 -8.5,3.75; P$4 -8.5,2.25; P$5 -8.5,0.75; P$6 -8.5,-0.75; P$7 -8.5,-2.25; P$8 -8.5,-3.75; P$9 -8.5,-5.25; P$10 -8.5,-6.75; P$11 8.5,-6.75; P$12 8.5,0.75; P$13 8.5,6.75 | hole 3: 0.5,0.85
FGPMMOPA6H = smd 2 x 1: P$1 -7.5,6.75; P$2 -7.5,5.25; P$3 -7.5,3.75; P$4 -7.5,2.25; P$5 -7.5,0.75; P$6 -7.5,-0.75; P$7 -7.5,-2.25; P$8 -7.5,-3.75; P$9 -7.5,-5.25; P$10 -7.5,-6.75; P$11 7.5,-6.75; P$12 7.5,-5.25; P$13 7.5,-3.75; P$14 7.5,-2.25; P$15 7.5,-0.75; P$16 7.5,0.75; P$17 7.5,2.25; P$18 7.5,3.75; P$19 7.5,5.25; P$20 7.5,6.75 | hole 3: 0.5,0.85
FH26-17S-0.3SHW = smd 0.3 x 0.8: 1 -2.4,-1.4; 2 -2.1,1.4; 3 -1.8,-1.4; 4 -1.5,1.4; 5 -1.2,-1.4; 6 -0.9,1.4; 7 -0.6,-1.4; 8 -0.3,1.4; 9 0,-1.4; 10 0.3,1.4; 11 0.6,-1.4; 12 0.9,1.4; 13 1.2,-1.4; 14 1.5,1.4; 15 1.8,-1.4; 16 2.1,1.4; 17 2.4,-1.4
FIDUCIAL-1.5X3 = smd 1.5 x 1.5: 1 0,0
FIDUCIAL-1X2 = smd 1 x 1: 1 0,0
FIDUCIAL-1X2.5 = smd 1 x 1: 1 0,0
FIDUCIAL_1MM = smd 1 x 1: 1 0,0
FPC4PIN = smd 0.26 x 1.4: 1 -0.75,0.15; 2 -0.25,0.15; 3 0.25,0.15; 4 0.75,0.15 | smd 2.45 x 2.6: GND1 -2.825,-1.565; GND2 2.83,-1.565
FPC40PIN = smd 0.275 x 1.5: P$1 -9.75,0.75; P$2 -9.25,0.75; P$3 -8.75,0.75; P$4 -8.25,0.75; P$5 -7.75,0.75; P$6 -7.25,0.75; P$7 -6.75,0.75; P$8 -6.25,0.75; P$9 -5.75,0.75; P$10 -5.25,0.75; P$11 -4.75,0.75; P$12 -4.25,0.75; P$13 -3.75,0.75; P$14 -3.25,0.75; P$15 -2.75,0.75; P$16 -2.25,0.75; P$17 -1.75,0.75; P$18 -1.25,0.75; P$19 -0.75,0.75; P$20 -0.25,0.75; P$21 0.25,0.75; P$22 0.75,0.75; P$23 1.25,0.75; P$24 1.75,0.75; P$25 2.25,0.75; P$26 2.75,0.75; P$27 3.25,0.75; P$28 3.75,0.75; P$29 4.25,0.75; P$30 4.75,0.75; P$31 5.25,0.75; P$32 5.75,0.75; P$33 6.25,0.75; P$34 6.75,0.75; P$35 7.25,0.75; P$36 7.75,0.75; P$37 8.25,0.75; P$38 8.75,0.75; P$39 9.25,0.75; P$40 9.75,0.75 | smd 1.8 x 2.2: SUPPORT1 -11.7,-2.4; SUPPORT2 11.7,-2.4
FPC45PIN = smd 0.3 x 1.2: P$1 -11,0; P$2 -10.5,0; P$3 -10,0; P$4 -9.5,0; P$5 -9,0; P$6 -8.5,0; P$7 -8,0; P$8 -7.5,0; P$9 -7,0; P$10 -6.5,0; P$11 -6,0; P$12 -5.5,0; P$13 -5,0; P$14 -4.5,0; P$15 -4,0; P$16 -3.5,0; P$17 -3,0; P$18 -2.5,0; P$19 -2,0; P$20 -1.5,0; P$21 -1,0; P$22 -0.5,0; P$23 0,0; P$24 0.5,0; P$25 1,0; P$26 1.5,0; P$27 2,0; P$28 2.5,0; P$29 3,0; P$30 3.5,0; P$31 4,0; P$32 4.5,0; P$33 5,0; P$34 5.5,0; P$35 6,0; P$36 6.5,0; P$37 7,0; P$38 7.5,0; P$39 8,0; P$40 8.5,0; P$41 9,0; P$42 9.5,0; P$43 10,0; P$44 10.5,0; P$45 11,0 | smd 2.4 x 2.4: P$46 -13.1,-2.7; P$47 13.1,-2.7
FPC_10PIN_52892-1095 = smd 0.25 x 1.4: P$1 -2.25,0; P$2 -1.75,0; P$3 -1.25,0; P$4 -0.75,0; P$5 -0.25,0; P$6 0.25,0; P$7 0.75,0; P$8 1.25,0; P$9 1.75,0; P$10 2.25,0 | smd 1.6 x 2.2: SUPPORT1 -4.9,-3.15; SUPPORT2 4.9,-3.15
FPC_XF2M-3015-1A = smd 0.25 x 1.1: P$1 7.25,-2.63; P$2 6.75,-2.63; P$3 6.25,-2.63; P$4 5.75,-2.63; P$5 5.25,-2.63; P$6 4.75,-2.63; P$7 4.25,-2.63; P$8 3.75,-2.63; P$9 3.25,-2.63; P$10 2.75,-2.63; P$11 2.25,-2.63; P$12 1.75,-2.63; P$13 1.25,-2.63; P$14 0.75,-2.63; P$15 0.25,-2.63; P$16 -0.25,-2.63; P$17 -0.75,-2.63; P$18 -1.25,-2.63; P$19 -1.75,-2.63; P$20 -2.25,-2.63; P$21 -2.75,-2.63; P$22 -3.25,-2.63; P$23 -3.75,-2.63; P$24 -4.25,-2.63; P$25 -4.75,-2.63; P$26 -5.25,-2.63; P$27 -5.75,-2.63; P$28 -6.25,-2.63; P$29 -6.75,-2.63; P$30 -7.25,-2.63 | smd 1.7 x 1.5: SUPPORT1 8.9,1.27; SUPPORT2 -8.9,1.27
GE864 = smd 1 x 1: A1 0,25; A2 0,22.5; A3 0,20; A4 0,17.5; A5 0,15; A6 0,12.5; A7 0,10; A8 0,7.5; A9 0,5; A10 0,2.5; A11 0,0; B1 2.5,25; B2 2.5,22.5; B3 2.5,20; B4 2.5,17.5; B5 2.5,15; B6 2.5,12.5; B7 2.5,10; B8 2.5,7.5; B9 2.5,5; B10 2.5,2.5; B11 2.5,0; C1 5,25; C2 5,22.5; C3 5,20; C4 5,17.5; C5 5,15; C6 5,12.5; C7 5,10; C8 5,7.5; C9 5,5; C10 5,2.5; C11 5,0; D1 7.5,25; D2 7.5,22.5; D3 7.5,20; D4 7.5,17.5; D5 7.5,15; D6 7.5,12.5; D7 7.5,10; D8 7.5,7.5; D9 7.5,5; D10 7.5,2.5; D11 7.5,0; E1 10,25; E2 10,22.5; E3 10,20; E4 10,17.5; E5 10,15; E6 10,12.5; E7 10,10; E8 10,7.5; E9 10,5; E10 10,2.5; E11 10,0; F1 12.5,25; F2 12.5,22.5; F3 12.5,20; F4 12.5,17.5; F5 12.5,15; F6 12.5,12.5; F7 12.5,10; F8 12.5,7.5; F9 12.5,5; F10 12.5,2.5; F11 12.5,0; G1 15,25; G2 15,22.5; G3 15,20; G4 15,17.5; G5 15,15; G6 15,12.5; G7 15,10; G8 15,7.5; G9 15,5; G10 15,2.5; G11 15,0; H1 17.5,25; H2 17.5,22.5; H3 17.5,20; H4 17.5,17.5; H5 17.5,15; H6 17.5,12.5; H7 17.5,10; H8 17.5,7.5; H9 17.5,5; H10 17.5,2.5; H11 17.5,0; J1 20,25; J2 20,22.5; J3 20,20; J4 20,17.5; J5 20,15; J6 20,12.5; J7 20,10; J8 20,7.5; J9 20,5; J10 20,2.5; J11 20,0; K1 22.5,25; K2 22.5,22.5; K3 22.5,20; K4 22.5,17.5; K5 22.5,15; K6 22.5,12.5; K7 22.5,10; K8 22.5,7.5; K9 22.5,5; K10 22.5,2.5; K11 22.5,0; L1 25,25; L2 25,22.5; L3 25,20; L4 25,17.5; L5 25,15; L6 25,12.5; L7 25,10; L8 25,7.5; L9 25,5; L10 25,2.5; L11 25,0
GE865 = smd 1 x 1: A1 -8.4,8.4; A2 -8.4,6; A3 -8.4,3.6; A4 -8.4,1.2; A5 -8.4,-1.2; A6 -8.4,-3.6; A7 -8.4,-6; A8 -8.4,-8.4; B1 -6,8.4; B2 -6,6; B3 -6,3.6; B4 -6,1.2; B5 -6,-1.2; B6 -6,-3.6; B7 -6,-6; B8 -6,-8.4; C1 -3.6,8.4; C2 -3.6,6; C3 -3.6,3.6; C4 -3.6,1.2; C5 -3.6,-1.2; C6 -3.6,-3.6; C7 -3.6,-6; C8 -3.6,-8.4; D1 -1.2,8.4; D2 -1.2,6; D3 -1.2,3.6; D4 -1.2,1.2; D5 -1.2,-1.2; D6 -1.2,-3.6; D7 -1.2,-6; D8 -1.2,-8.4; E1 1.2,8.4; E2 1.2,6; E3 1.2,3.6; E4 1.2,1.2; E5 1.2,-1.2; E6 1.2,-3.6; E7 1.2,-6; E8 1.2,-8.4; F1 3.6,8.4; F2 3.6,6; F3 3.6,3.6; F4 3.6,1.2; F5 3.6,-1.2; F6 3.6,-3.6; F7 3.6,-6; F8 3.6,-8.4; G1 6,8.4; G2 6,6; G3 6,3.6; G4 6,1.2; G5 6,-1.2; G6 6,-3.6; G7 6,-6; G8 6,-8.4; H1 8.4,8.4; H2 8.4,6; H3 8.4,3.6; H4 8.4,1.2; H5 8.4,-1.2; H6 8.4,-3.6; H7 8.4,-6; H8 8.4,-8.4
GM862 = smd 1.2 x 0.25: 1 -12.898,3.791; 2 -16.298,3.794; 3 -12.898,4.291; 4 -16.298,4.294; 5 -12.898,4.791; 6 -16.298,4.794; 7 -12.898,5.291; 8 -16.298,5.294; 9 -12.898,5.791; 10 -16.298,5.794; 11 -12.899,6.29; 12 -16.298,6.294; 13 -12.898,6.791; 14 -16.298,6.794; 15 -12.898,7.291; 16 -16.298,7.294; 17 -12.898,7.791; 18 -16.298,7.794; 19 -12.898,8.291; 20 -16.298,8.294; 21 -12.898,8.791; 22 -16.298,8.794; 23 -12.898,9.291; 24 -16.298,9.294; 25 -12.898,9.791; 26 -16.298,9.794; 27 -12.898,10.291; 28 -16.298,10.294; 29 -12.898,10.791; 30 -16.298,10.794; 31 -12.898,11.291; 32 -16.298,11.294; 33 -12.898,11.791; 34 -16.298,11.794; 35 -12.898,12.291; 36 -16.298,12.294; 37 -12.898,12.791; 38 -16.298,12.794; 39 -12.898,13.291; 40 -16.298,13.294; 41 -12.898,13.791; 42 -16.298,13.794; 43 -12.898,14.291; 44 -16.298,14.294; 45 -12.898,14.791; 46 -16.298,14.794; 47 -12.898,15.291; 48 -16.298,15.294; 49 -12.898,15.791; 50 -16.298,15.794 | drill 1.2: G1 -10,21.5; G2 0,21.5; G3 10,21.5; G4 21.5,0; G5 10,-21.5; G6 0,-21.5; G7 -10,-21.5; G8 -21.5,0
GM862_CONNECTOR = smd 1.2 x 0.25: 1 1.707,-6.016; 2 -1.693,-6.013; 3 1.707,-5.516; 4 -1.693,-5.513; 5 1.707,-5.016; 6 -1.693,-5.013; 7 1.707,-4.516; 8 -1.693,-4.513; 9 1.707,-4.016; 10 -1.693,-4.013; 11 1.706,-3.517; 12 -1.693,-3.513; 13 1.707,-3.016; 14 -1.693,-3.013; 15 1.707,-2.516; 16 -1.693,-2.513; 17 1.707,-2.016; 18 -1.693,-2.013; 19 1.707,-1.516; 20 -1.693,-1.513; 21 1.707,-1.016; 22 -1.693,-1.013; 23 1.707,-0.516; 24 -1.693,-0.513; 25 1.707,-0.016; 26 -1.693,-0.013; 27 1.707,0.484; 28 -1.693,0.487; 29 1.707,0.984; 30 -1.693,0.987; 31 1.707,1.484; 32 -1.693,1.487; 33 1.707,1.984; 34 -1.693,1.987; 35 1.707,2.484; 36 -1.693,2.487; 37 1.707,2.984; 38 -1.693,2.987; 39 1.707,3.484; 40 -1.693,3.487; 41 1.707,3.984; 42 -1.693,3.987; 43 1.707,4.484; 44 -1.693,4.487; 45 1.707,4.984; 46 -1.693,4.987; 47 1.707,5.484; 48 -1.693,5.487; 49 1.707,5.984; 50 -1.693,5.987 | drill 0.025 pad 0.025: G1 0,-11.43; G2 0,-11.43; G3 0,-11.43; G4 0,-11.43; G5 0,-11.43; G6 0,-11.43; G7 0,-11.43; G8 0,-11.43
HB100 = drill 1.5: 5V@1 -17.81,15.83; 5V@2 -20.35,15.83; GND@1 17.81,15.83; GND@2 15.27,15.83; GND@3 20.35,-18.37; GND@4 17.81,-18.37; IF@1 -17.81,-18.37; IF@2 -20.35,-18.37
HC49UP = smd 5.334 x 1.93: 1 -4.826,0; 2 4.826,0
HDMI_MOLEX_47151-0001 = smd 0.3 x 2.6: 1 4.5,0; 2 4,0; 3 3.5,0; 4 3,0; 5 2.5,0; 6 2,0; 7 1.5,0; 8 1,0; 9 0.5,0; 10 0,0; 11 -0.5,0; 12 -1,0; 13 -1.5,0; 14 -2,0; 15 -2.5,0; 16 -3,0; 17 -3.5,0; 18 -4,0; 19 -4.5,0 | drill 0.9 pad 1.65 long: P$1 -7.25,-0.76; P$2 7.25,-0.76 | drill 0.9 pad 1.5 long: P$3 7.25,-6.72; P$4 -7.25,-6.72
HEADER_1X02 = drill 1 square: 1 0,0 | drill 1: 2 2.54,0
HEADER_1X05 = drill 1 square: 1 0,0 | drill 1: 2 2.54,0; 3 5.08,0; 4 7.62,0; 5 10.16,0
HMC5883L = smd 0.45 x 0.26: 1 -1.275,0.75; 2 -1.275,0.25; 3 -1.275,-0.25; 4 -1.275,-0.75; 9 1.275,-0.75; 10 1.275,-0.25; 11 1.275,0.25; 12 1.275,0.75 | smd 0.26 x 0.45: 5 -0.75,-1.275; 6 -0.25,-1.275; 7 0.25,-1.275; 8 0.75,-1.275; 13 0.75,1.275; 14 0.25,1.275; 15 -0.25,1.275; 16 -0.75,1.275
HMC5883L_EXTENDED = smd 0.95 x 0.26: 1 -1.525,0.75; 2 -1.525,0.25; 3 -1.525,-0.25; 4 -1.525,-0.75; 9 1.525,-0.75; 10 1.525,-0.25; 11 1.525,0.25; 12 1.525,0.75 | smd 0.26 x 0.95: 5 -0.75,-1.525; 6 -0.25,-1.525; 7 0.25,-1.525; 8 0.75,-1.525; 13 0.75,1.525; 14 0.25,1.525; 15 -0.25,1.525; 16 -0.75,1.525
HTSSOP16 = smd 0.3 x 1.6: P$1 -2.275,-2.8; P$2 -1.625,-2.8; P$3 -0.975,-2.8; P$4 -0.325,-2.8; P$5 0.325,-2.8; P$6 0.975,-2.8; P$7 1.625,-2.8; P$8 2.275,-2.8; P$9 2.275,2.8; P$10 1.625,2.8; P$11 0.975,2.8; P$12 0.325,2.8; P$13 -0.325,2.8; P$14 -0.975,2.8; P$15 -1.625,2.8; P$16 -2.275,2.8 | smd 4.8 x 3.2: P$17 0,0
HVQFN32 = smd 0.9 x 0.3: 1 -2.5,1.75; 2 -2.5,1.25; 3 -2.5,0.75; 4 -2.5,0.25; 5 -2.5,-0.25; 6 -2.5,-0.75; 7 -2.5,-1.25; 8 -2.5,-1.75; 17 2.5,-1.75; 18 2.5,-1.25; 19 2.5,-0.75; 20 2.5,-0.25; 21 2.5,0.25; 22 2.5,0.75; 23 2.5,1.25; 24 2.5,1.75 | smd 0.3 x 0.9: 9 -1.75,-2.5; 10 -1.25,-2.5; 11 -0.75,-2.5; 12 -0.25,-2.5; 13 0.25,-2.5; 14 0.75,-2.5; 15 1.25,-2.5; 16 1.75,-2.5; 25 1.75,2.5; 26 1.25,2.5; 27 0.75,2.5; 28 0.25,2.5; 29 -0.25,2.5; 30 -0.75,2.5; 31 -1.25,2.5; 32 -1.75,2.5 | smd 0.7 x 0.7: DNC(FIDUCIAL) -3.127,3.127 | smd 3.2 x 3.2: PAD 0,0
HVQFN32-5X5 = smd 1.1 x 0.25: 1 -2.55,1.75; 2 -2.55,1.25; 3 -2.55,0.75; 4 -2.55,0.25; 5 -2.55,-0.25; 6 -2.55,-0.75; 7 -2.55,-1.25; 8 -2.55,-1.75; 17 2.55,-1.75; 18 2.55,-1.25; 19 2.55,-0.75; 20 2.55,-0.25; 21 2.55,0.25; 22 2.55,0.75; 23 2.55,1.25; 24 2.55,1.75 | smd 0.25 x 1.1: 9 -1.75,-2.55; 10 -1.25,-2.55; 11 -0.75,-2.55; 12 -0.25,-2.55; 13 0.25,-2.55; 14 0.75,-2.55; 15 1.25,-2.55; 16 1.75,-2.55; 25 1.75,2.55; 26 1.25,2.55; 27 0.75,2.55; 28 0.25,2.55; 29 -0.25,2.55; 30 -0.75,2.55; 31 -1.25,2.55; 32 -1.75,2.55
HVQFN32-5X5_3MMTHERMAL = smd 1.1 x 0.25: 1 -2.55,1.75; 2 -2.55,1.25; 3 -2.55,0.75; 4 -2.55,0.25; 5 -2.55,-0.25; 6 -2.55,-0.75; 7 -2.55,-1.25; 8 -2.55,-1.75; 17 2.55,-1.75; 18 2.55,-1.25; 19 2.55,-0.75; 20 2.55,-0.25; 21 2.55,0.25; 22 2.55,0.75; 23 2.55,1.25; 24 2.55,1.75 | smd 0.25 x 1.1: 9 -1.75,-2.55; 10 -1.25,-2.55; 11 -0.75,-2.55; 12 -0.25,-2.55; 13 0.25,-2.55; 14 0.75,-2.55; 15 1.25,-2.55; 16 1.75,-2.55; 25 1.75,2.55; 26 1.25,2.55; 27 0.75,2.55; 28 0.25,2.55; 29 -0.25,2.55; 30 -0.75,2.55; 31 -1.25,2.55; 32 -1.75,2.55 | smd 3 x 3: THERMAL 0,0
HVQFN33-7X7 = smd 1.067 x 0.3: P$1 -3.327,2.275; P$2 -3.327,1.625; P$3 -3.327,0.975; P$4 -3.327,0.325; P$5 -3.327,-0.325; P$6 -3.327,-0.975; P$7 -3.327,-1.625; P$8 -3.327,-2.275; P$17 3.327,-2.275; P$18 3.327,-1.625; P$19 3.327,-0.975; P$20 3.327,-0.325; P$21 3.327,0.325; P$22 3.327,0.975; P$23 3.327,1.625; P$24 3.327,2.275 | smd 0.3 x 1.067: P$9 -2.275,-3.327; P$10 -1.625,-3.327; P$11 -0.975,-3.327; P$12 -0.325,-3.327; P$13 0.325,-3.327; P$14 0.975,-3.327; P$15 1.625,-3.327; P$16 2.275,-3.327; P$25 2.275,3.327; P$26 1.625,3.327; P$27 0.975,3.327; P$28 0.325,3.327; P$29 -0.325,3.327; P$30 -0.975,3.327; P$31 -1.625,3.327; P$32 -2.275,3.327 | smd 4 x 4: P$33 0,0
HVQFN40-6X6 = smd 1 x 0.25: 1 -2.99,2.25; 2 -2.99,1.75; 3 -2.99,1.25; 4 -2.99,0.75; 5 -2.99,0.25; 6 -2.99,-0.25; 7 -2.99,-0.75; 8 -2.99,-1.25; 9 -2.99,-1.75; 10 -2.99,-2.25; 21 2.99,-2.25; 22 2.99,-1.75; 23 2.99,-1.25; 24 2.99,-0.75; 25 2.99,-0.25; 26 2.99,0.25; 27 2.99,0.75; 28 2.99,1.25; 29 2.99,1.75; 30 2.99,2.25 | smd 0.25 x 1: 11 -2.25,-2.99; 12 -1.75,-2.99; 13 -1.25,-2.99; 14 -0.75,-2.99; 15 -0.25,-2.99; 16 0.25,-2.99; 17 0.75,-2.99; 18 1.25,-2.99; 19 1.75,-2.99; 20 2.25,-2.99; 31 2.25,2.99; 32 1.75,2.99; 33 1.25,2.99; 34 0.75,2.99; 35 0.25,2.99; 36 -0.25,2.99; 37 -0.75,2.99; 38 -1.25,2.99; 39 -1.75,2.99; 40 -2.25,2.99 | smd 4 x 4: TP 0,0
HVQFN64 = smd 0.9 x 0.3: 1 -4.6,3.75; 2 -4.6,3.25; 3 -4.6,2.75; 4 -4.6,2.25; 5 -4.6,1.75; 6 -4.6,1.25; 7 -4.6,0.75; 8 -4.6,0.25; 9 -4.6,-0.25; 10 -4.6,-0.75; 11 -4.6,-1.25; 12 -4.6,-1.75; 13 -4.6,-2.25; 14 -4.6,-2.75; 15 -4.6,-3.25; 16 -4.6,-3.75; 33 4.6,-3.75; 34 4.6,-3.25; 35 4.6,-2.75; 36 4.6,-2.25; 37 4.6,-1.75; 38 4.6,-1.25; 39 4.6,-0.75; 40 4.6,-0.25; 41 4.6,0.25; 42 4.6,0.75; 43 4.6,1.25; 44 4.6,1.75; 45 4.6,2.25; 46 4.6,2.75; 47 4.6,3.25; 48 4.6,3.75 | smd 0.3 x 0.9: 17 -3.75,-4.6; 18 -3.25,-4.6; 19 -2.75,-4.6; 20 -2.25,-4.6; 21 -1.75,-4.6; 22 -1.25,-4.6; 23 -0.75,-4.6; 24 -0.25,-4.6; 25 0.25,-4.6; 26 0.75,-4.6; 27 1.25,-4.6; 28 1.75,-4.6; 29 2.25,-4.6; 30 2.75,-4.6; 31 3.25,-4.6; 32 3.75,-4.6; 49 3.75,4.6; 50 3.25,4.6; 51 2.75,4.6; 52 2.25,4.6; 53 1.75,4.6; 54 1.25,4.6; 55 0.75,4.6; 56 0.25,4.6; 57 -0.25,4.6; 58 -0.75,4.6; 59 -1.25,4.6; 60 -1.75,4.6; 61 -2.25,4.6; 62 -2.75,4.6; 63 -3.25,4.6; 64 -3.75,4.6 | smd 0.7 x 0.7: P$1 -5.85,5.85 | smd 5.1 x 5.1: PAD 0,0
ILI9325_28INCH_TS = smd 0.5 x 2: 1 -18,0; 2 -17,0; 3 -16,0; 4 -15,0; 5 -14,0; 6 -13,0; 7 -12,0; 8 -11,0; 9 -10,0; 10 -9,0; 11 -8,0; 12 -7,0; 13 -6,0; 14 -5,0; 15 -4,0; 16 -3,0; 17 -2,0; 18 -1,0; 19 0,0; 20 1,0; 21 2,0; 22 3,0; 23 4,0; 24 5,0; 25 6,0; 26 7,0; 27 8,0; 28 9,0; 29 10,0; 30 11,0; 31 12,0; 32 13,0; 33 14,0; 34 15,0; 35 16,0; 36 17,0; 37 18,0 | hole 1: -19.5,0; 19.5,0
ILI9325_28INCH_TS_OUTLINE = smd 0.5 x 3: 1 -18,27.77; 2 -17,27.77; 3 -16,27.77; 4 -15,27.77; 5 -14,27.77; 6 -13,27.77; 7 -12,27.77; 8 -11,27.77; 9 -10,27.77; 10 -9,27.77; 11 -8,27.77; 12 -7,27.77; 13 -6,27.77; 14 -5,27.77; 15 -4,27.77; 16 -3,27.77; 17 -2,27.77; 18 -1,27.77; 19 0,27.77; 20 1,27.77; 21 2,27.77; 22 3,27.77; 23 4,27.77; 24 5,27.77; 25 6,27.77; 26 7,27.77; 27 8,27.77; 28 9,27.77; 29 10,27.77; 30 11,27.77; 31 12,27.77; 32 13,27.77; 33 14,27.77; 34 15,27.77; 35 16,27.77; 36 17,27.77; 37 18,27.77
ILI9481_35INCH_OUTLINE = smd 0.5 x 3 bottom: 1 -18,48.57; 2 -17,48.57; 3 -16,48.57; 4 -15,48.57; 5 -14,48.57; 6 -13,48.57; 7 -12,48.57; 8 -11,48.57; 9 -10,48.57; 10 -9,48.57; 11 -8,48.57; 12 -7,48.57; 13 -6,48.57; 14 -5,48.57; 15 -4,48.57; 16 -3,48.57; 17 -2,48.57; 18 -1,48.57; 19 0,48.57; 20 1,48.57; 21 2,48.57; 22 3,48.57; 23 4,48.57; 24 5,48.57; 25 6,48.57; 26 7,48.57; 27 8,48.57; 28 9,48.57; 29 10,48.57; 30 11,48.57; 31 12,48.57; 32 13,48.57; 33 14,48.57; 34 15,48.57; 35 16,48.57; 36 17,48.57; 37 18,48.57
INDUCTOR_5X5MM_NR5040_NOTHERMALS = smd 1.8 x 4: P$1 -1.8,0; P$2 1.8,0
INDUCTOR_5X5MM_TDK_VLC5045 = smd 2.54 x 5: P$1 -2.096,0; P$2 2.096,0
INDUCTOR_5X5MM_TDK_VLC5045_NOTHERMALS = smd 2.54 x 5: P$1 -2.096,0; P$2 2.096,0
INDUCTOR_6X6MM_TDK_SLF6045 = smd 1.5 x 2.2: P$1 -2.75,0; P$2 2.75,0
INDUCTOR_6X6MM_TDK_VLC6045 = smd 3.25 x 6: P$1 -2.35,0; P$2 2.35,0
INDUCTOR_1007 = smd 1.016 x 2.2: P$1 -1.127,0; P$2 1.127,0
ITG3200_QFN24 = smd 0.8 x 0.28: 1 -2,1.25; 2 -2,0.75; 3 -2,0.25; 4 -2,-0.25; 5 -2,-0.75; 6 -2,-1.25; 13 2,-1.25; 14 2,-0.75; 15 2,-0.25; 16 2,0.25; 17 2,0.75; 18 2,1.25 | smd 0.28 x 0.8: 7 -1.25,-2; 8 -0.75,-2; 9 -0.25,-2; 10 0.25,-2; 11 0.75,-2; 12 1.25,-2; 19 1.25,2; 20 0.75,2; 21 0.25,2; 22 -0.25,2; 23 -0.75,2; 24 -1.25,2 | smd 1.778 x 1.778: THERM 0,0
JD-T1800 = smd 0.5 x 2: 1 5.2,-13.1; 2 4.4,-13.1; 3 3.6,-13.1; 4 2.8,-13.1; 5 2,-13.1; 6 1.2,-13.1; 7 0.4,-13.1; 8 -0.4,-13.1; 9 -1.2,-13.1; 10 -2,-13.1; 11 -2.8,-13.1; 12 -3.6,-13.1; 13 -4.4,-13.1; 14 -5.2,-13.1 | hole 0.6: -12.8,-16.9; 7.65,-16.9
JSTPH2 = smd 1 x 4.6: 1 -1,-3.7; 2 1,-3.7 | smd 1.6 x 3.4: NC1 -3.4,1.5; NC2 3.4,1.5
JSTPH2_NOTHERMALS = smd 1 x 4.6: 1 -1,-3.7; 2 1,-3.7 | smd 1.6 x 3.4: NC1 -3.4,1.5; NC2 3.4,1.5
JSTPH3 = smd 1 x 4.6: 1 -2,-2.7; 2 0,-2.7; 3 2,-2.7 | smd 1.6 x 3.4: NC1 -4.4,2.5; NC2 4.4,2.5
JSTPH4 = smd 1 x 4.6: 1 -3,-3.7; 2 -1,-3.7; 3 1,-3.7; 4 3,-3.7 | smd 1.7 x 3.4: NC1 -5.7,1.5; NC2 5.7,1.5
JSTPH6 = smd 1 x 4.6: 1 -5,-3.7; 2 -3,-3.7; 3 -1,-3.7; 4 1,-3.7; 5 3,-3.7; 6 5,-3.7 | smd 1.7 x 3.4: NC1 -7.7,1.5; NC2 7.7,1.5
JSTPH8 = smd 1 x 4.6: 1 -7,-3.7; 2 -5,-3.7; 3 -3,-3.7; 4 -1,-3.7; 5 1,-3.7; 6 3,-3.7; 7 5,-3.7; 8 7,-3.7 | smd 1.7 x 3.4: NC1 -9.7,1.5; NC2 9.7,1.5
JSTSH2 = smd 0.5 x 1.35: 1 -0.5,-2.55; 2 0.5,-2.55 | smd 1.2 x 2: NC1 -1.8,1.125; NC2 1.8,1.125
JTAG-ARM = drill 1: 1 -11.43,-1.27 | drill 1 octagon: 2 -11.43,1.27; 3 -8.89,-1.27; 4 -8.89,1.27; 5 -6.35,-1.27; 6 -6.35,1.27; 7 -3.81,-1.27; 8 -3.81,1.27; 9 -1.27,-1.27; 10 -1.27,1.27; 11 1.27,-1.27; 12 1.27,1.27; 13 3.81,-1.27; 14 3.81,1.27; 15 6.35,-1.27; 16 6.35,1.27; 17 8.89,-1.27; 18 8.89,1.27; 19 11.43,-1.27; 20 11.43,1.27
JUMPER2 = drill 1 pad 1.93 octagon: 1 2.54,0; 2 0,0
JUMPER3 = drill 1 pad 1.93 octagon: 1 -2.54,0; 2 0,0; 3 2.54,0
L3G4200D_LGA16L = smd 0.6 x 0.3: P$1 -1.6,0.975; P$2 -1.6,0.325; P$3 -1.6,-0.325; P$4 -1.6,-0.975; P$9 1.6,-0.975; P$10 1.6,-0.325; P$11 1.6,0.325; P$12 1.6,0.975 | smd 0.3 x 0.6: P$5 -0.975,-1.6; P$6 -0.325,-1.6; P$7 0.325,-1.6; P$8 0.975,-1.6; P$13 0.975,1.6; P$14 0.325,1.6; P$15 -0.325,1.6; P$16 -0.975,1.6
LBGA256_1.0MM = smd 0.45 x 0.45: A1 -7.5,7.5; A2 -6.5,7.5; A3 -5.5,7.5; A4 -4.5,7.5; A5 -3.5,7.5; A6 -2.5,7.5; A7 -1.5,7.5; A8 -0.5,7.5; A9 0.5,7.5; A10 1.5,7.5; A11 2.5,7.5; A12 3.5,7.5; A13 4.5,7.5; A14 5.5,7.5; A15 6.5,7.5; A16 7.5,7.5; B1 -7.5,6.5; B2 -6.5,6.5; B3 -5.5,6.5; B4 -4.5,6.5; B5 -3.5,6.5; B6 -2.5,6.5; B7 -1.5,6.5; B8 -0.5,6.5; B9 0.5,6.5; B10 1.5,6.5; B11 2.5,6.5; B12 3.5,6.5; B13 4.5,6.5; B14 5.5,6.5; B15 6.5,6.5; B16 7.5,6.5; C1 -7.5,5.5; C2 -6.5,5.5; C3 -5.5,5.5; C4 -4.5,5.5; C5 -3.5,5.5; C6 -2.5,5.5; C7 -1.5,5.5; C8 -0.5,5.5; C9 0.5,5.5; C10 1.5,5.5; C11 2.5,5.5; C12 3.5,5.5; C13 4.5,5.5; C14 5.5,5.5; C15 6.5,5.5; C16 7.5,5.5; D1 -7.5,4.5; D2 -6.5,4.5; D3 -5.5,4.5; D4 -4.5,4.5; D5 -3.5,4.5; D6 -2.5,4.5; D7 -1.5,4.5; D8 -0.5,4.5; D9 0.5,4.5; D10 1.5,4.5; D11 2.5,4.5; D12 3.5,4.5; D13 4.5,4.5; D14 5.5,4.5; D15 6.5,4.5; D16 7.5,4.5; E1 -7.5,3.5; E2 -6.5,3.5; E3 -5.5,3.5; E4 -4.5,3.5; E5 -3.5,3.5; E6 -2.5,3.5; E7 -1.5,3.5; E8 -0.5,3.5; E9 0.5,3.5; E10 1.5,3.5; E11 2.5,3.5; E12 3.5,3.5; E13 4.5,3.5; E14 5.5,3.5; E15 6.5,3.5; E16 7.5,3.5; F1 -7.5,2.5; F2 -6.5,2.5; F3 -5.5,2.5; F4 -4.5,2.5; F5 -3.5,2.5; F6 -2.5,2.5; F7 -1.5,2.5; F8 -0.5,2.5; F9 0.5,2.5; F10 1.5,2.5; F11 2.5,2.5; F12 3.5,2.5; F13 4.5,2.5; F14 5.5,2.5; F15 6.5,2.5; F16 7.5,2.5; G1 -7.5,1.5; G2 -6.5,1.5; G3 -5.5,1.5; G4 -4.5,1.5; G5 -3.5,1.5; G6 -2.5,1.5; G7 -1.5,1.5; G8 -0.5,1.5; G9 0.5,1.5; G10 1.5,1.5; G11 2.5,1.5; G12 3.5,1.5; G13 4.5,1.5; G14 5.5,1.5; G15 6.5,1.5; G16 7.5,1.5; H1 -7.5,0.5; H2 -6.5,0.5; H3 -5.5,0.5; H4 -4.5,0.5; H5 -3.5,0.5; H6 -2.5,0.5; H7 -1.5,0.5; H8 -0.5,0.5; H9 0.5,0.5; H10 1.5,0.5; H11 2.5,0.5; H12 3.5,0.5; H13 4.5,0.5; H14 5.5,0.5; H15 6.5,0.5; H16 7.5,0.5; J1 -7.5,-0.5; J2 -6.5,-0.5; J3 -5.5,-0.5; J4 -4.5,-0.5; J5 -3.5,-0.5; J6 -2.5,-0.5; J7 -1.5,-0.5; J8 -0.5,-0.5; J9 0.5,-0.5; J10 1.5,-0.5; J11 2.5,-0.5; J12 3.5,-0.5; J13 4.5,-0.5; J14 5.5,-0.5; J15 6.5,-0.5; J16 7.5,-0.5; K1 -7.5,-1.5; K2 -6.5,-1.5; K3 -5.5,-1.5; K4 -4.5,-1.5; K5 -3.5,-1.5; K6 -2.5,-1.5; K7 -1.5,-1.5; K8 -0.5,-1.5; K9 0.5,-1.5; K10 1.5,-1.5; K11 2.5,-1.5; K12 3.5,-1.5; K13 4.5,-1.5; K14 5.5,-1.5; K15 6.5,-1.5; K16 7.5,-1.5; L1 -7.5,-2.5; L2 -6.5,-2.5; L3 -5.5,-2.5; L4 -4.5,-2.5; L5 -3.5,-2.5; L6 -2.5,-2.5; L7 -1.5,-2.5; L8 -0.5,-2.5; L9 0.5,-2.5; L10 1.5,-2.5; L11 2.5,-2.5; L12 3.5,-2.5; L13 4.5,-2.5; L14 5.5,-2.5; L15 6.5,-2.5; L16 7.5,-2.5; M1 -7.5,-3.5; M2 -6.5,-3.5; M3 -5.5,-3.5; M4 -4.5,-3.5; M5 -3.5,-3.5; M6 -2.5,-3.5; M7 -1.5,-3.5; M8 -0.5,-3.5; M9 0.5,-3.5; M10 1.5,-3.5; M11 2.5,-3.5; M12 3.5,-3.5; M13 4.5,-3.5; M14 5.5,-3.5; M15 6.5,-3.5; M16 7.5,-3.5; N1 -7.5,-4.5; N2 -6.5,-4.5; N3 -5.5,-4.5; N4 -4.5,-4.5; N5 -3.5,-4.5; N6 -2.5,-4.5; N7 -1.5,-4.5; N8 -0.5,-4.5; N9 0.5,-4.5; N10 1.5,-4.5; N11 2.5,-4.5; N12 3.5,-4.5; N13 4.5,-4.5; N14 5.5,-4.5; N15 6.5,-4.5; N16 7.5,-4.5; P1 -7.5,-5.5; P2 -6.5,-5.5; P3 -5.5,-5.5; P4 -4.5,-5.5; P5 -3.5,-5.5; P6 -2.5,-5.5; P7 -1.5,-5.5; P8 -0.5,-5.5; P9 0.5,-5.5; P10 1.5,-5.5; P11 2.5,-5.5; P12 3.5,-5.5; P13 4.5,-5.5; P14 5.5,-5.5; P15 6.5,-5.5; P16 7.5,-5.5; R1 -7.5,-6.5; R2 -6.5,-6.5; R3 -5.5,-6.5; R4 -4.5,-6.5; R5 -3.5,-6.5; R6 -2.5,-6.5; R7 -1.5,-6.5; R8 -0.5,-6.5; R9 0.5,-6.5; R10 1.5,-6.5; R11 2.5,-6.5; R12 3.5,-6.5; R13 4.5,-6.5; R14 5.5,-6.5; R15 6.5,-6.5; R16 7.5,-6.5; T1 -7.5,-7.5; T2 -6.5,-7.5; T3 -5.5,-7.5; T4 -4.5,-7.5; T5 -3.5,-7.5; T6 -2.5,-7.5; T7 -1.5,-7.5; T8 -0.5,-7.5; T9 0.5,-7.5; T10 1.5,-7.5; T11 2.5,-7.5; T12 3.5,-7.5; T13 4.5,-7.5; T14 5.5,-7.5; T15 6.5,-7.5; T16 7.5,-7.5 | smd 0.7 x 0.7: FIDUCIAL -8.89,8.89
LFCSP16-R = smd 1.9 x 1.9: 0 0,0 | smd 0.65 x 0.35: 1 -1.75,0.975; 2 -1.75,0.325; 3 -1.75,-0.325; 4 -1.75,-0.975; 9 1.75,-0.975; 10 1.75,-0.325; 11 1.75,0.325; 12 1.75,0.975 | smd 0.35 x 0.65: 5 -0.975,-1.75; 6 -0.325,-1.75; 7 0.325,-1.75; 8 0.975,-1.75; 13 0.975,1.75; 14 0.325,1.75; 15 -0.325,1.75; 16 -0.975,1.75
LFCSP16-W = smd 1.9 x 1.9: 0 0,0 | smd 1.558 x 0.35: 1 -2.204,0.975; 2 -2.204,0.325; 3 -2.204,-0.325; 4 -2.204,-0.975; 9 2.204,-0.975; 10 2.204,-0.325; 11 2.204,0.325; 12 2.204,0.975 | smd 0.35 x 1.558: 5 -0.975,-2.204; 6 -0.325,-2.204; 7 0.325,-2.204; 8 0.975,-2.204; 13 0.975,2.204; 14 0.325,2.204; 15 -0.325,2.204; 16 -0.975,2.204
LGA8 = smd 1.9 x 0.6: P$1 -1.5,1.875; P$2 -1.5,0.625; P$3 -1.5,-0.625; P$4 -1.5,-1.875; P$5 1.5,-1.875; P$6 1.5,-0.625; P$7 1.5,0.625; P$8 1.5,1.875
LGA14 = smd 0.5 x 1.2: 1 2,1.1; 2 1.2,1.1; 3 0.4,1.1; 4 -0.4,1.1; 5 -1.2,1.1; 6 -2,1.1; 8 -2,-1.1; 9 -1.2,-1.1; 10 -0.4,-1.1; 11 0.4,-1.1; 12 1.2,-1.1; 13 2,-1.1 | smd 1.2 x 0.5: 7 -2.1,0; 14 2.1,0
LGA16_3X3MM = smd 0.8 x 0.25: 1 -1.45,1; 2 -1.45,0.5; 3 -1.45,0; 4 -1.45,-0.5; 5 -1.45,-1; 9 1.45,-1; 10 1.45,-0.5; 11 1.45,0; 12 1.45,0.5; 13 1.45,1 | smd 0.25 x 0.8: 6 -0.5,-1.45; 7 0,-1.45; 8 0.5,-1.45; 14 0.5,1.45; 15 0,1.45; 16 -0.5,1.45
LGA16_5X5MM = smd 1.2 x 0.5: 1 -2.3,1.6; 2 -2.3,0.8; 3 -2.3,0; 4 -2.3,-0.8; 5 -2.3,-1.6; 9 2.3,-1.6; 10 2.3,-0.8; 11 2.3,0; 12 2.3,0.8; 13 2.3,1.6 | smd 0.5 x 1.2: 6 -0.8,-2.3; 7 0,-2.3; 8 0.8,-2.3; 14 0.8,2.3; 15 0,2.3; 16 -0.8,2.3
LLP40 = smd 0.25 x 0.6: 1 2.25,2.9; 2 1.75,2.9; 3 1.25,2.9; 4 0.75,2.9; 5 0.25,2.9; 6 -0.25,2.9; 7 -0.75,2.9; 8 -1.25,2.9; 9 -1.75,2.9; 10 -2.25,2.9; 21 -2.25,-2.9; 22 -1.75,-2.9; 23 -1.25,-2.9; 24 -0.75,-2.9; 25 -0.25,-2.9; 26 0.25,-2.9; 27 0.75,-2.9; 28 1.25,-2.9; 29 1.75,-2.9; 30 2.25,-2.9 | smd 0.6 x 0.25: 11 -2.9,2.25; 12 -2.9,1.75; 13 -2.9,1.25; 14 -2.9,0.75; 15 -2.9,0.25; 16 -2.9,-0.25; 17 -2.9,-0.75; 18 -2.9,-1.25; 19 -2.9,-1.75; 20 -2.9,-2.25; 31 2.9,-2.25; 32 2.9,-1.75; 33 2.9,-1.25; 34 2.9,-0.75; 35 2.9,-0.25; 36 2.9,0.25; 37 2.9,0.75; 38 2.9,1.25; 39 2.9,1.75; 40 2.9,2.25 | smd 4.3 x 4.3: 41 0,0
